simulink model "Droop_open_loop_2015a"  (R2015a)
settings: Solver=ode23tb  SolverMode=SingleTasking  StartTime=0.0  StopTime=4  RelTol=1e-4
undefined symbols (not defined in the file): D1, Delta
libraries: powerlib x12, powerlib_meascontrol x1

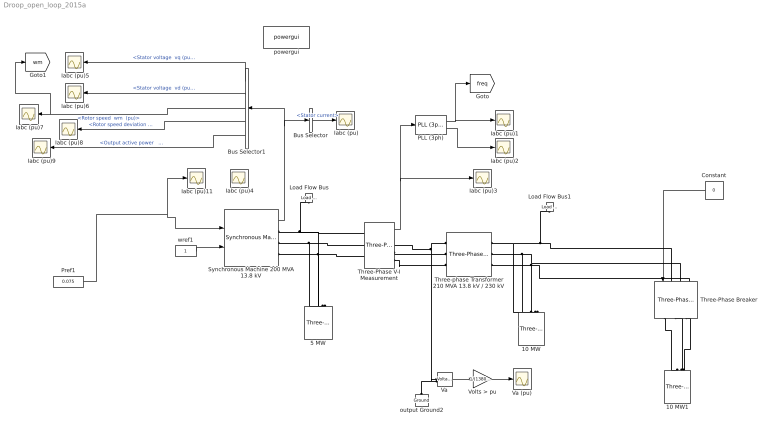
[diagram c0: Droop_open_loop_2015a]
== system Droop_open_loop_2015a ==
   Iabc (pu){,1..9,11} (11 alike) : Scope
  10 MW : powerlib/Elements/Three-Phase Parallel RLC Load  LConnTagsString=A|B|C  Configuration=Y (grounded)  NominalVoltage=230e3  Vabc=[1e3 1e3 1e3]  Vabcp=[1e3 1e3 1e3]  NominalFrequency=60  UnbalancedPower=off  ActivePower=10000000  InductivePower=0  CapacitivePower=0  Pabc=[10e3 9e3 11e3]  QLabc=[100 90 110]  QCabc=[100 90 110]  Pabcp=[10e3 9e3 11e3]  QLabcp=[100 90 110]  QCabcp=[100 90 110]  Measurements=None  LoadType=constant Z
  10 MW1 : powerlib/Elements/Three-Phase Parallel RLC Load  LConnTagsString=A|B|C  Configuration=Y (grounded)  NominalVoltage=230e3  Vabc=[1e3 1e3 1e3]  Vabcp=[1e3 1e3 1e3]  NominalFrequency=60  UnbalancedPower=off  ActivePower=10000000  InductivePower=0  CapacitivePower=0  Pabc=[10e3 9e3 11e3]  QLabc=[100 90 110]  QCabc=[100 90 110]  Pabcp=[10e3 9e3 11e3]  QLabcp=[100 90 110]  QCabcp=[100 90 110]  Measurements=None  LoadType=constant Z
  5 MW : powerlib/Elements/Three-Phase Parallel RLC Load  LConnTagsString=A|B|C  Configuration=Y (grounded)  NominalVoltage=13.8e3  Vabc=[1e3 1e3 1e3]  Vabcp=[1e3 1e3 1e3]  NominalFrequency=60  UnbalancedPower=off  ActivePower=5000000  InductivePower=0  CapacitivePower=0  Pabc=[10e3 9e3 11e3]  QLabc=[100 90 110]  QCabc=[100 90 110]  Pabcp=[10e3 9e3 11e3]  QLabcp=[100 90 110]  QCabcp=[100 90 110]  Measurements=None  LoadType=constant Z
  Bus Selector : BusSelector  OutputSignals=Stator current
  Bus Selector1 : BusSelector  OutputSignals="dq0 components.Stator voltage  vq (pu),dq0 components.Stator voltage  vd (pu),Mechanical.Rotor speed  wm  (pu),Mechanical.Rotor speed deviation  dw (pu),Output active power   Peo (pu)"
  Constant : Constant  Value=0
  Load Flow Bus : powerlib/Measurements/Load Flow Bus  LConnTagsString=a  Phases=single  Connectors=on one side  ID=B1  Vbase=13.8e3  Vref=1  Vangle=0  VLF=1  VLFb=1  VLFc=1  angleLF=-23.67  angleLFb=0  angleLFc=0
  Load Flow Bus1 : powerlib/Measurements/Load Flow Bus  LConnTagsString=a  Phases=single  Connectors=on one side  ID=B2  Vbase=230e3  Vref=1  Vangle=0  VLF=1  VLFb=1  VLFc=1  angleLF=0  angleLFb=0  angleLFc=0
  PLL (3ph) : powerlib_meascontrol/PLL/PLL (3ph)  Fmin=45  Par_Init=[0, 60]  ParK=[180, 3200, 1]  TcD=1e-4  MaxRateChangeFreq=12  FilterCutOffFreq=25  Ts=0  AGC=on
  Pref1 : Constant  Value=0.075
  Synchronous Machine 200 MVA 13.8 kV : powerlib/Machines/Synchronous Machine pu Standard  PresetModel=No  MechanicalLoad=Mechanical power Pm  ShowDetailedParameters=on  RotorType=Salient-pole  Units=per unit standard parameters  MeasurementBus=off  NominalParameters="[ 200E6  13800   60 ]"  Reactances1=[ 31 32 33 34 35 36 37 ]  Reactances2=[ 1.305, 0.296, 0.252, 0.474, 0.243, 0.18 ]  dAxisTimeConstants=Short-circuit  qAxisTimeConstants=Open-circuit  TimeConstants1=[]  TimeConstants2=[]  TimeConstants3=[]  TimeConstants4=[]  TimeConstants5=[ 1.01, 0.053, 0.1 ]  TimeConstants6=[]  TimeConstants7=[]  TimeConstants8=[]  StatorResistance=2.8544e-3  Mechanical=[ 3.2 0 2]  PolePairs=2  InitialConditions=[0 -94.2826 0.750185 0.750185 0.750185 -24.943 -144.943 95.057 1.29071]  SetSaturation=off  Saturation=[0.6404,0.7127,0.8441,0.9214,0.9956,1.082,1.19,1.316,1.457;0.7,0.7698,0.8872,0.9466,0.9969,1.046,1.1,1.151,1.201]  LoadFlowParameters=[1 150000000 0 0]  TsPowergui=0  TsBlock=-1  IterativeModel=Trapezoidal non iterative  IterativeDiscreteModel=Trapezoidal non iterative  BusType=PV  Pref=150000000  Qref=0  Qmin=-Inf  Qmax=Inf  PLF=0  QLF=0
  Three-Phase V-I Measurement : powerlib/Measurements/Three-Phase V-I Measurement  VoltageMeasurement=phase-to-ground  SetLabelV=off  LabelV=Vabc  Vpu=off  VpuLL=off  CurrentMeasurement=yes  SetLabelI=off  LabelI=Iabc  Ipu=off  Pbase=100e6  Vbase=500e3  OutputType=Complex  PhasorSimulation=off  PSBequivalent=0
  Three-Phase Breaker : powerlib/Elements/Three-Phase Breaker  InitialState=open  SwitchA=on  SwitchB=on  SwitchC=on  SwitchTimes="[30/60  60/60]"  External=on  BreakerResistance=0.01  SnubberResistance=1e6  SnubberCapacitance=inf  Measurements=None
  Three-phase Transformer 210 MVA 13.8 kV / 230 kV : powerlib/Elements/Three-Phase Transformer (Two Windings)  Winding1Connection=Delta (D1)  Winding2Connection=Yg  CoreType=Three single-phase transformers  SetSaturation=off  Hysteresis=off  DataFile='hysteresis'  SetInitialFlux=off  Measurements=None  UNITS=pu  NominalPower=[ 210e6 60 ]  Winding1="[ 13.8e3 0.0027  0.08]"  Winding2=[ 230e3 0.0027 0.08]  Rm=500  Lm=500  L0=0.5  Saturation="[ 0,0  ;  0.005,1.2  ;  1.0,1.4 ]"  InitialFluxes=[ 0.8 , -0.8 , 0.7 ]  MoreParameters=off  BreakLoop=off  DataType=off  TransfoNumber=0
  Va : powerlib/Measurements/Voltage Measurement  Tag=PoWeRsYsTeMmEaSuReMeNt  PhasorSimulation=off  OutputType=Magnitude  PSBequivalent=0
  Va (pu) : Scope
  Volts > pu : Gain  Gain=1/(13800/sqrt(3)*sqrt(2))
  output Ground2 : powerlib/Elements/Ground  LConnTagsString=a
  powergui : powerlib/powergui  Priority=2  SimulationMode=Continuous  SampleTime=0  frequency=60  Iterations=50  frequencyindice=60  Pbase=100e6  ErrMax=0.0001  UnitsV=kV  UnitsW=MW  buscounter=0  FunctionMessages=off  echomessages=off  EnableUseOfTLC=off  CurrentSourceSwitches=off  DisableSnubberDevices=off  DisableRonSwitches=off  DisableVfSwitches=off  DisplayEquations=off  SolverType=Tustin  Interpol=off  ExternalGateDelay=off  methode=off  Ts=0  x0status=blocks  SPID=on  SwTol=0  HookPort=off  RestoreLinks=warning  ResistiveCurrentMeasurement=off  Frange=logspace(0,3,50)  Ylog=off  Xlog=off  ShowGrid=off  save=off  variable=ZData  structure=0  ZoomFFT=on  StartTime=0.0  cycles=2  DisplayStyle=off  fundamental=60  FreqAxis=off  MaxFrequency=1000  frequencyindicesteady=1  RmsSteady=1  display=off
  wref1 : Constant
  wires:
  Volts > pu/1 -> Va (pu)/1
  Synchronous Machine 200 MVA 13.8 kV/1 -> Bus Selector/1, Bus Selector1/1
  Va/1 -> Volts > pu/1
  Bus Selector/1 -> " Iabc (pu)"/1  "<Stator current>"
  Three-Phase V-I Measurement/1 -> " Iabc (pu)3"/1, PLL (3ph)/1
  PLL (3ph)/1 -> [freq], " Iabc (pu)1"/1
  PLL (3ph)/2 -> " Iabc (pu)2"/1
  Constant/1 -> Three-Phase Breaker/1
  wref1/1 -> Synchronous Machine 200 MVA 13.8 kV/2
  Bus Selector1/5 -> " Iabc (pu)9"/1  "<Output active power   Peo (pu)>"
  Bus Selector1/4 -> " Iabc (pu)8"/1  "<Rotor speed deviation  dw (pu)>"
  Bus Selector1/3 -> [wm], " Iabc (pu)7"/1  "<Rotor speed  wm  (pu)>"
  Bus Selector1/2 -> " Iabc (pu)6"/1  "<Stator voltage  vd (pu)>"
  Bus Selector1/1 -> " Iabc (pu)5"/1  "<Stator voltage  vq (pu)>"
  Pref1/1 -> Synchronous Machine 200 MVA 13.8 kV/1, " Iabc (pu)11"/1
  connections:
  output Ground2/LConn1 -- Va/LConn2
  Synchronous Machine 200 MVA 13.8 kV/RConn3 -- 5 MW/LConn3 -- Three-Phase V-I Measurement/LConn3
  Synchronous Machine 200 MVA 13.8 kV/RConn2 -- 5 MW/LConn2 -- Three-Phase V-I Measurement/LConn2
  Synchronous Machine 200 MVA 13.8 kV/RConn1 -- Three-Phase V-I Measurement/LConn1 -- 5 MW/LConn1 -- Load Flow Bus/LConn1
  Three-phase Transformer 210 MVA 13.8 kV / 230 kV/RConn1 -- Three-Phase Breaker/LConn1 -- Load Flow Bus1/LConn1 -- 10 MW/LConn1
  Three-phase Transformer 210 MVA 13.8 kV / 230 kV/LConn1 -- Va/LConn1 -- Three-Phase V-I Measurement/RConn1
  Three-Phase V-I Measurement/RConn2 -- Three-phase Transformer 210 MVA 13.8 kV / 230 kV/LConn2
  Three-Phase V-I Measurement/RConn3 -- Three-phase Transformer 210 MVA 13.8 kV / 230 kV/LConn3
  Three-phase Transformer 210 MVA 13.8 kV / 230 kV/RConn2 -- Three-Phase Breaker/LConn2 -- 10 MW/LConn2
  Three-phase Transformer 210 MVA 13.8 kV / 230 kV/RConn3 -- Three-Phase Breaker/LConn3 -- 10 MW/LConn3
  Three-Phase Breaker/RConn1 -- 10 MW1/LConn1
  10 MW1/LConn2 -- Three-Phase Breaker/RConn2
  10 MW1/LConn3 -- Three-Phase Breaker/RConn3
